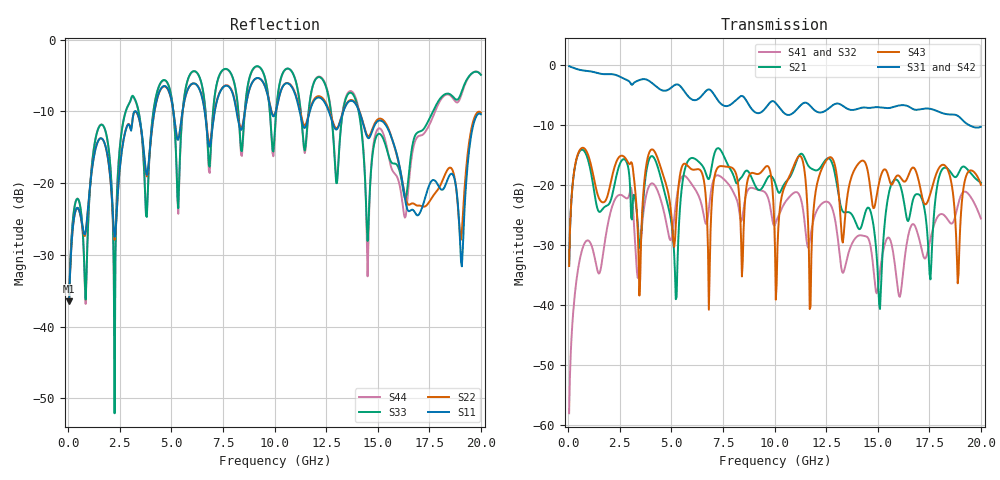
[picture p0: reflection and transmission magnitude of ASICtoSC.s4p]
! Touchstone generated by fitter/viewer
# HZ S  RI R 5.000000e+001
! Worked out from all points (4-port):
!   499 points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, 40.08 MHz to 20 GHz, reference 50 ohm
!   strongest paths, dB at 40.08 MHz, 5.01 GHz, 10.02 GHz, 15.03 GHz, 20 GHz:
!     S31: -0.1, -3.7, -6.2, -7.0, -10.3
!     S42: -0.1, -3.7, -6.2, -7.1, -10.4
!     S43: -33.5, -25.6, -30.6, -20.2, -19.9
!     S21: -33.5, -26.5, -19.6, -36.8, -19.6
!     S41: -58.0, -28.8, -26.6, -36.6, -25.5
!     S32: -58.0, -28.9, -26.8, -36.5, -25.9
!   lowest |S11| = -36.5 dB at 40.08 MHz (marker M1), VSWR 1.03, Z = 51.3 - j0.752 ohm
!   |S11| at or under -10 dB: start of sweep to 3.215 GHz; 3.281 GHz to 4.173 GHz (892.6 MHz wide, 23.9 % of centre); 14.1 GHz to end of sweep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
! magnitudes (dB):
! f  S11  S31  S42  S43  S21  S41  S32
! 40.08 MHz  -36.5  -0.1  -0.1  -33.5  -33.5  -58.0  -58.0
! 2.445 GHz  -19.7  -1.8  -1.8  -15.4  -17.0  -21.7  -21.6
! 11.74 GHz  -9.6  -6.8  -6.9  -40.2  -17.1  -28.4  -28.7
! 12.63 GHz  -10.0  -7.2  -7.3  -15.4  -15.5  -22.9  -23.0
! 15.11 GHz  -11.3  -7.0  -7.1  -18.9  -40.6  -34.3  -34.3
! 19.08 GHz  -31.6  -9.0  -9.0  -22.8  -17.0  -21.4  -21.6
! 20 GHz  -10.4  -10.3  -10.4  -19.9  -19.6  -25.5  -25.9
